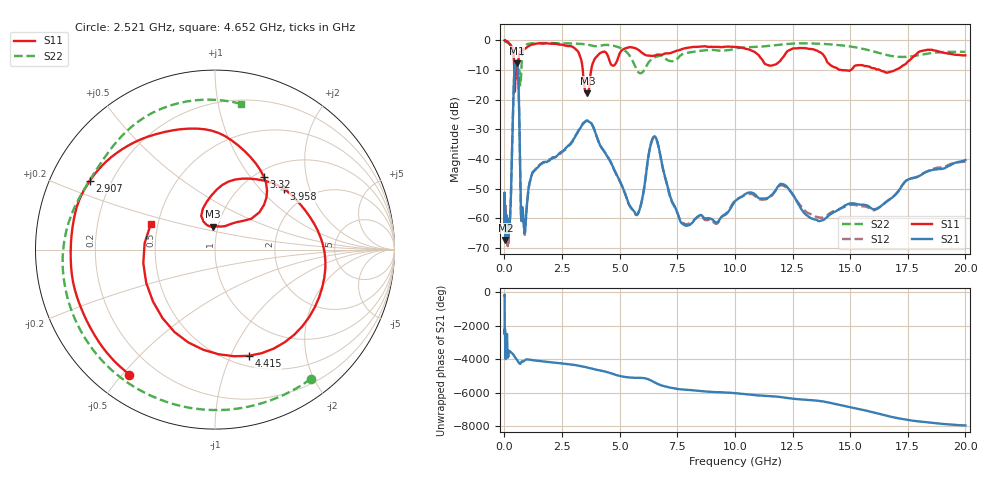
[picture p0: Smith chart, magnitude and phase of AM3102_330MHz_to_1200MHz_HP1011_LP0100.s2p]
! Date/Time: Tue, Sep 11, 2018 5:20 PM
! Network Analyzer: Agilent Technologies E8362B Rev: A.07.50.63
! Sweep from 0.010 to 20.000 GHz, 1601 Points, Sweep Type: LOG
! Power Supply: 4.949 V, 0.001 A
# Hz S DB R 50
!freq MagS11 AngS11 MagS21 AngS21 MagS12 AngS12 MagS22 AngS22
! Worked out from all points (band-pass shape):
!   1601 points, 10 MHz to 20 GHz, reference 50 ohm
!   highest |S21| = -7.69 dB at 535.7 MHz (marker M1); lowest = -67.3 dB at 41.59 MHz (marker M2)
!   |S21| within 3 dB of the highest: 431 MHz to 592.7 MHz (161.7 MHz wide, 31.6 % of centre)
!   lowest |S11| = -17.8 dB at 3.599 GHz (marker M3), VSWR 1.30, Z = 47.3 + j12.3 ohm
!   |S11| at or under -10 dB: 3.402 GHz to 3.765 GHz (362.8 MHz wide, 10.1 % of centre); 14.66 GHz to 15.02 GHz (364.3 MHz wide, 2.45 % of centre); 16.3 GHz to 16.95 GHz (658.1 MHz wide, 3.96 % of centre)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
!   |S22| runs from -15.1 to -0.2 dB; largest |S21 - S12| = 0.0054
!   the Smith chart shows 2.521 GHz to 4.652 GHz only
!   S11 on the Smith chart (normalised r, x): 2.521 GHz: 0.11, -0.52; 2.907 GHz: 0.12, +0.25; 3.32 GHz: 1.09, +1.17; 3.958 GHz: 1.49, +1.37; 4.415 GHz: 0.61, -1.17; 4.652 GHz: 0.46, +0.15
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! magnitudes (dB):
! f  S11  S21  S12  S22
! 10 MHz  0.0  -51.6  -56.2  -0.2
! 35.55 MHz  0.0  -63.1  -65.0  -0.3
! 41.59 MHz  0.0  -67.3  -65.3  -0.3
! 126.4 MHz  -0.4  -64.6  -64.9  -0.7
! 244.6 MHz  -1.2  -59.1  -60.4  -1.5
! 447.2 MHz  -16.8  -8.9  -9.0  -6.3
! 535.7 MHz  -8.0  -7.7  -7.7  -8.1
! 617.7 MHz  -5.8  -16.0  -16.0  -10.6
! 726 MHz  -3.4  -59.8  -59.4  -11.7
! 869.7 MHz  -2.9  -64.6  -65.1  -2.0
! 1.59 GHz  -1.0  -41.6  -41.6  -0.9
! 2.521 GHz  -1.5  -37.3  -37.4  -1.0
! 2.907 GHz  -2.0  -34.5  -34.3  -1.0
! 3.32 GHz  -6.2  -29.2  -29.2  -1.1
! 3.599 GHz  -17.8  -27.1  -27.0  -1.4
! 3.958 GHz  -5.8  -31.4  -31.3  -2.0
! 4.415 GHz  -4.1  -38.4  -38.3  -1.5
! 4.652 GHz  -8.3  -41.6  -41.7  -1.7
! 5.652 GHz  -2.5  -57.9  -58.1  -8.4
! 6.487 GHz  -5.2  -32.4  -32.6  -5.8
! 7.92 GHz  -2.5  -62.4  -61.9  -4.2
! 20 GHz  -5.0  -40.3  -40.9  -3.8
